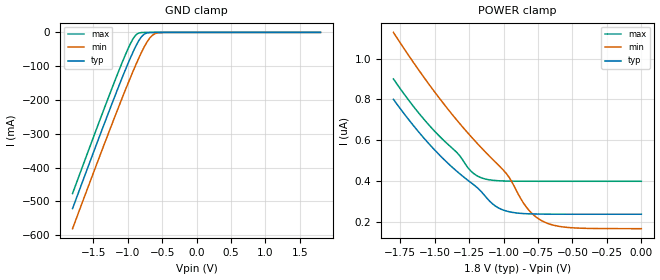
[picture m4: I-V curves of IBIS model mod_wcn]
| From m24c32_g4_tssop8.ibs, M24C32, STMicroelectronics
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|   Model mod_wcn
[Model]   mod_wcn
Model_type Input
Vinl   =   0.540V
Vinh   =   1.260V
C_comp   2.193pF   2.023pF   2.323pF
[Temperature Range]  25.0000   0.1050k   -40.0000
[Voltage Range]   1.8000V   1.7000V   2.0000V
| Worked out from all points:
|   GND clamp passes 1 mA (typ) near -0.70 V on its own axis
[GND_clamp]
|Voltage   I(typ)   I(min)   I(max)
-1.8V     -520.9mA   -580.4mA   -476.5mA
-1.2V     -196.3mA   -256.7mA   -150.7mA
-1.04V    -114.2mA   -173.9mA   -69.64mA
-960mV    -75.5mA    -133.8mA   -33.45mA
-880mV    -40.19mA   -95.31mA   -7.265mA
-800mV    -12.93mA   -59.48mA   -440.5uA
-760mV    -5.12mA    -43.24mA   -160.1uA
-720mV    -1.577mA   -28.79mA   -103.5uA
-640mV    -137.4uA   -8.393mA   -71.39uA
-560mV    -29.54uA   -1.293mA   -48.43uA
-480mV    -12.59uA   -165.5uA   -27.66uA
1.8V      235.7nA    165nA      397.6nA
[POWER_clamp]
|Voltage   I(typ)   I(min)   I(max)
-1.8V     800.1nA    1.129uA    900.3nA
-1.5V     550.9nA    835.6nA    642.8nA
-1.34V    446.9nA    698.3nA    539.3nA
-1.22V    382nA      604.6nA    436.9nA
-1.14V    329.5nA    546.7nA    409.9nA
-1.02V    261.1nA    465nA      399.6nA
-960mV    248nA      416.9nA    398.4nA
-840mV    238.4nA    275.2nA    397.7nA
-760mV    236.7nA    219.7nA    397.7nA
-660mV    235.9nA    186.1nA    397.6nA
-540mV    235.7nA    171.2nA    397.6nA
0V        235.7nA    164.9nA    397.6nA
